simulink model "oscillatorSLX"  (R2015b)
settings: Solver=VariableStepAuto  StartTime=0.0  StopTime=10.0  RelTol=1e-3
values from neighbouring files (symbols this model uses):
  D = 0.02    [oscillator.m]    (also in oscillator_simulink.m)
  Ekin = 10    [oscillator.m]    (also in oscillator_simulink.m)
  k = 20    [oscillator.m]    (also in oscillator_simulink.m)
  m = 1    [oscillator.m]    (also in oscillator_simulink.m)

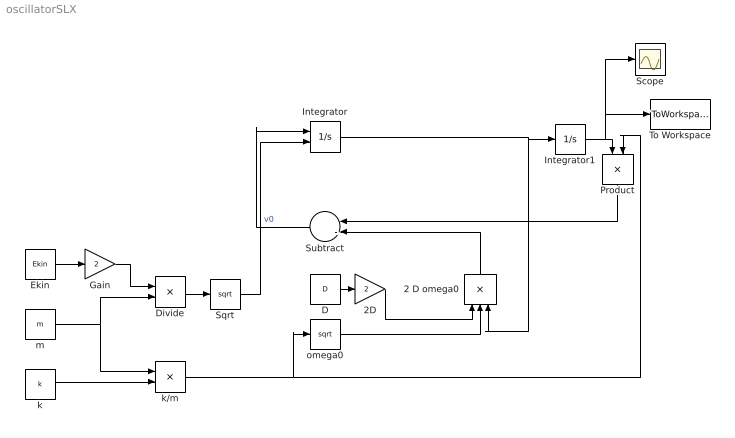
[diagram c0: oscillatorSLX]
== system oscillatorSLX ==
  2 D omega0 : Product  Inputs=3
  2D : Gain  Gain=2
  D : Constant  Value=D
  Divide : Product  Inputs=*/
  Ekin : Constant  Value=Ekin
  Gain : Gain  Gain=2
  Integrator : Integrator  InitialConditionSource=external
  Integrator1 : Integrator
  Product : Product
  Scope : Scope
  Sqrt : Sqrt
  Subtract : Sum  Inputs=--
  To Workspace : ToWorkspace  VariableName=simulation  SaveFormat=Timeseries  SampleTime=-1
  k : Constant  Value=k
  k/m : Product  Inputs=/*
  m : Constant  Value=m
  omega0 : Sqrt
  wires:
  Integrator/1 -> 2 D omega0/3, Integrator1/1
  Ekin/1 -> Gain/1
  Gain/1 -> Divide/1
  m/1 -> Divide/2, k/m/1
  Divide/1 -> Sqrt/1
  Sqrt/1 -> Integrator/2  "v0"
  Subtract/1 -> Integrator/1
  k/1 -> k/m/2
  Integrator1/1 -> To Workspace/1, Scope/1, Product/1
  Product/1 -> Subtract/1
  k/m/1 -> omega0/1, Product/2
  D/1 -> 2D/1
  omega0/1 -> 2 D omega0/2
  2D/1 -> 2 D omega0/1
  2 D omega0/1 -> Subtract/2
